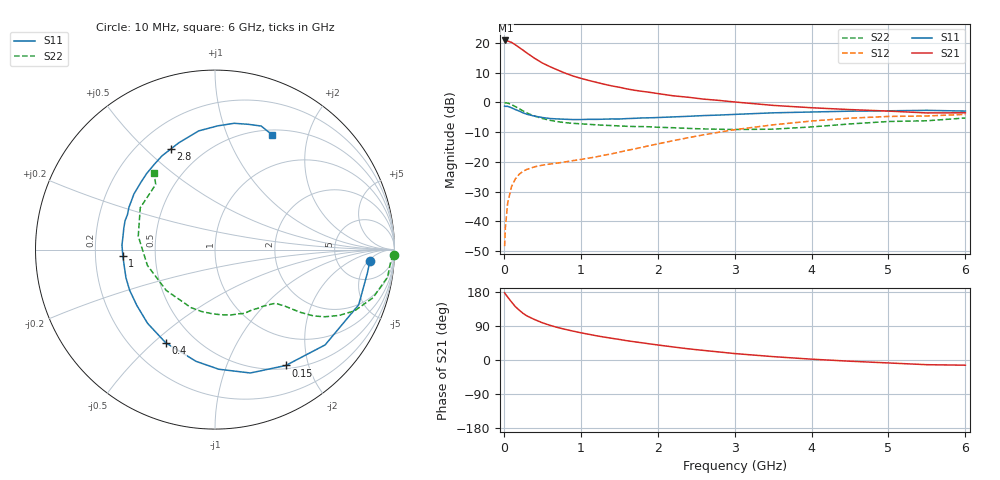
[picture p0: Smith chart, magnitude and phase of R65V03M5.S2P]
! SIEMENS Small Signal Semiconductors
! BFR193
! Si NPN RF Bipolar Junction Transistor in SOT23
! VCE = 5 V  IC = 3.5 mA
! Common Emitter S-Parameters:  May  1996
# GHz  S  MA  R  50
!  f  S11  S21  S12  S22
! GHz  MAG  ANG  MAG  ANG  MAG  ANG  MAG  ANG
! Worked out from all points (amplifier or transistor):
!   36 points, 10 MHz to 6 GHz, reference 50 ohm
!   highest |S21| = 20.9 dB at 20 MHz (marker M1)
!   |S21| within 3 dB of that: start of sweep to 234.7 MHz
!   unconditionally stable (mu >= 1): 1.011 GHz to 2.024 GHz
!   at 250 MHz: K = 0.33, MSG = 20.4 dB, |S12| = -23.2 dB
!   at 1.4 GHz: K = 1.08, MAG = 9.7 dB, |S12| = -17.3 dB
!   at 6 GHz: K = 0.98, MSG = 0.3 dB, |S12| = -4.0 dB
!   S11 on the Smith chart (normalised r, x): 10 MHz: 11, -6; 150 MHz: 0.55, -1.65; 400 MHz: 0.35, -0.55; 1 GHz: 0.32, -0.03; 2.8 GHz: 0.34, +0.60; 6 GHz: 0.56, +1.46
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0.01  0.8651 -4.2  11.03 177.4  0.0038 87.7  0.9959 -1.7
0.02  0.8594 -8.5  11.04 174.2  0.0078 87.3  0.9822 -3.7
0.05  0.8577 -21.0  10.82 166.0  0.0204 78.9  0.9733 -9.1
0.1  0.8113 -40.9  10.24 153.0  0.0382 69.7  0.9199 -17.0
0.15  0.7565 -58.6  9.316 140.8  0.0516 61.2  0.849 -23.7
0.2  0.7151 -74.0  8.404 131.5  0.0619 54.8  0.7819 -28.0
0.25  0.6668 -88.2  7.566 123.1  0.0692 50.5  0.718 -31.4
0.3  0.6315 -99.6  6.784 116.4  0.0746 47.4  0.6634 -33.9
0.4  0.5872 -117.9  5.529 106.7  0.0824 43.4  0.5879 -36.4
0.5  0.5567 -132.4  4.61 98.3  0.0877 41.9  0.5366 -37.8
0.6  0.5354 -144.3  3.996 91.5  0.0917 42.1  0.4995 -39.0
0.7  0.5268 -154.7  3.507 85.7  0.0954 43.1  0.4741 -40.3
0.8  0.5202 -162.5  3.099 80.8  0.0997 44.5  0.4555 -41.3
1  0.5147 -176.1  2.545 71.9  0.1095 47.8  0.4356 -44.2
1.1  0.519 177.3  2.35 68.0  0.1151 50.0  0.4278 -46.3
1.6  0.5343 153.8  1.687 50.9  0.1554 57.9  0.3959 -57.7
2.2  0.5697 132.0  1.292 34.5  0.2267 59.6  0.3749 -76.5
2.8  0.6123 113.6  1.08 21.1  0.3155 54.6  0.3529 -102.4
3.5  0.6676 97.8  0.891 8.9  0.4194 43.6  0.3542 -139.9
4.5  0.7117 81.4  0.757 -3.2  0.5429 25.4  0.434 170.1
5.5  0.735 69.5  0.665 -12.4  0.5915 7.2  0.4908 132.3
6  0.7148 63.7  0.669 -13.7  0.6279 2.1  0.5467 128.4
